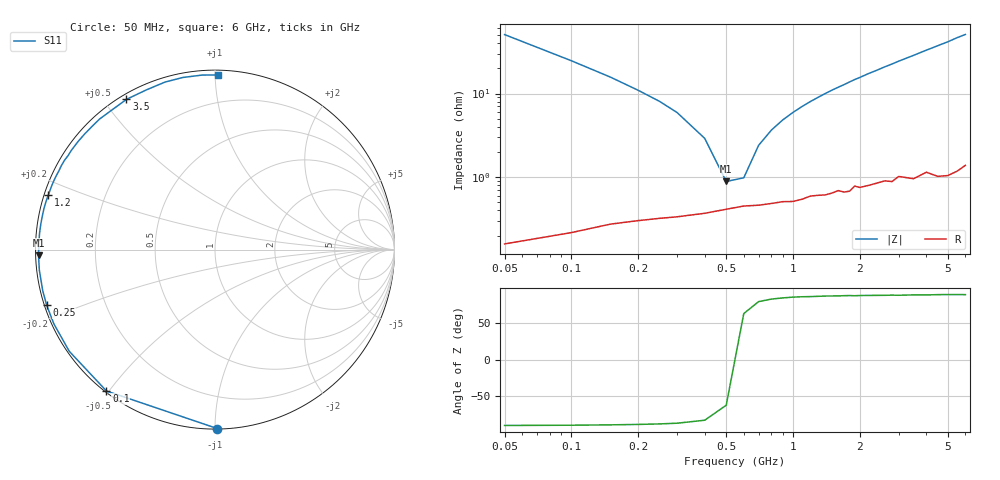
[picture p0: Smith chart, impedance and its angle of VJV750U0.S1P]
! Infineon Technologies  Discrete & RF Semiconductors
! BB 914
! Si Tuning Diode in SOT23
! VR = 0.75 V
! S-Parameters:  July  1999
# GHz  S  MA  R  50
!  f  S11
! GHz  MAG  ANG
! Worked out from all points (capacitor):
!   34 points, 50 MHz to 6 GHz, reference 50 ohm
!   read as one part to ground: C = 62.4 pF near 50 MHz
!   lowest |Z| = 888 mohm at 500 MHz (marker M1)
!   series resonance near 547.4 MHz, so ESL is about 1.4 nH
!   S11 on the Smith chart (normalised r, x): 50 MHz: 0.00, -1.01; 100 MHz: 0.00, -0.49; 250 MHz: 0.01, -0.16; 1.2 GHz: 0.01, +0.16; 3.5 GHz: 0.02, +0.57; 6 GHz: 0.03, +1.02
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0.05  0.9969 -89.3
0.1  0.993 -127.5
0.15  0.9901 -145.1
0.2  0.9885 -155.3
0.25  0.9875 -161.7
0.3  0.9868 -166.5
0.4  0.9854 -173.4
0.5  0.9836 -178.2
0.6  0.9821 178.0
0.7  0.9817 174.6
0.8  0.9809 171.7
1  0.98 166.5
1.2  0.9771 161.8
1.4  0.9767 157.4
1.6  0.9742 153.3
1.8  0.975 149.3
2  0.9729 145.5
2.2  0.9719 141.7
2.4  0.9707 138.3
2.6  0.9697 134.7
2.8  0.971 131.5
3  0.9675 128.1
3.5  0.9715 120.5
4  0.9685 113.2
4.5  0.9741 106.6
5  0.9756 100.6
5.5  0.975 94.2
6  0.9731 89.1
